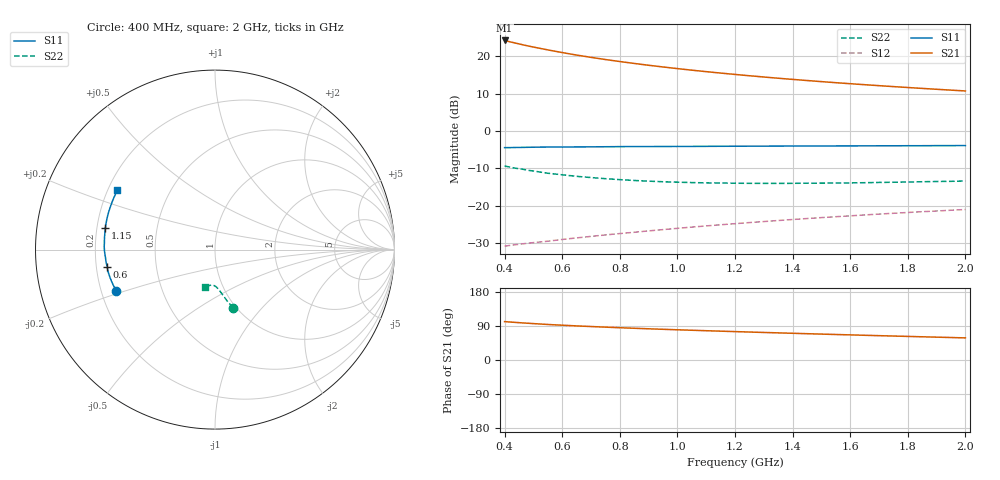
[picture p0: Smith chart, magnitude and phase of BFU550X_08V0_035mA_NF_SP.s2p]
! Filename:  P:\Prog\Test\Noise\ATS_data\Testdata_Net\BFU550X attenuator noise\BFU550X_APG2013_44_C05_08p0V_035mA_NF_CM01_D.sf
! Date/Time: Fri 26/Jul/2013 14:34:24
! BFU550X_APG2013_44_C05_08p0V_1to35mA_NF_CM01_Bias8_R.sf
! Noise Parameter Data File
! BFU550X_APG2013_44_C05_08p0V_1to35mA_NF_CM01
! Date/time: Mon Jul 22 10:19:05 2013
! VAR V_out= 8.001000
! VAR I_out= 34.995000
! VAR V_in= 0.782000
! VAR I_in= 0.370650
! Device data file deembeded for feedlines and parallel
! Original file: \BFU550X attenuator noise\BFU550X_APG2013_44_C05_08p0V_035mA_NF_CM01_R.sf
! Feed-files: PR005V01_100713_Feed1.s2p, PR005V01_100713_Feed2.s2p
! Parallel-file: PR005V01_100713_Par.s2p
# MHz S MA R 50
!  Freq-MHz  S11-mag  S11-arg  S21-mag  S21-arg  S12-mag  S12-arg  S22-mag  S22-arg
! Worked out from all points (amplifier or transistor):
!   37 points, 400 MHz to 2 GHz, reference 50 ohm
!   highest |S21| = 24.2 dB at 400 MHz (marker M1)
!   |S21| within 3 dB of that: start of sweep to 583.3 MHz
!   unconditionally stable (mu >= 1): 1.217 GHz to end of sweep
!   at 500 MHz: K = 0.74, MSG = 26.2 dB, |S12| = -29.9 dB
!   at 1.1 GHz: K = 0.98, MSG = 20.6 dB, |S12| = -25.4 dB
!   at 2 GHz: K = 1.05, MAG = 14.5 dB, |S12| = -21.0 dB
!   lowest NFmin = 1.31 dB at 480 MHz
!   S11 on the Smith chart (normalised r, x): 400 MHz: 0.26, -0.19; 600 MHz: 0.25, -0.07; 1.15 GHz: 0.23, +0.09; 2 GHz: 0.24, +0.27
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400  0.597 -157.4  16.2 101.3  0.02873 50.4  0.3391 -72.8
420  0.5974 -159.1  15.5 100.1  0.02947 50.8  0.3269 -73.9
440  0.6003 -160.7  14.87 99.1  0.03015 51.0  0.3158 -74.5
460  0.6017 -162.2  14.28 98.0  0.0308 51.3  0.3085 -75.6
480  0.6033 -163.6  13.72 97.0  0.03142 51.6  0.2978 -76.4
500  0.6053 -165.0  13.22 96.0  0.03205 51.9  0.2907 -77.0
550  0.6083 -168.4  12.12 93.7  0.03346 53.1  0.2715 -78.7
600  0.6082 -170.9  11.16 91.8  0.03531 53.9  0.2587 -80.1
650  0.6108 -173.4  10.34 90.0  0.03707 54.7  0.2469 -81.3
700  0.6116 -175.7  9.628 88.3  0.0388 55.5  0.2376 -82.6
750  0.614 -177.8  9.008 86.7  0.04062 56.2  0.2297 -83.7
800  0.6161 -179.7  8.467 85.2  0.04235 56.8  0.2228 -84.9
900  0.6173 176.6  7.548 82.4  0.04599 58.1  0.2127 -86.9
950  0.6187 174.9  7.163 81.0  0.04784 58.5  0.2089 -87.8
1050  0.6203 171.8  6.491 78.5  0.05169 59.4  0.2036 -89.6
1150  0.6226 169.0  5.935 76.1  0.05553 59.9  0.2009 -91.3
1200  0.6236 167.5  5.692 74.9  0.05742 60.1  0.1997 -92.2
1350  0.6264 163.5  5.064 71.6  0.06329 60.6  0.1985 -94.6
1500  0.6288 159.8  4.562 68.4  0.06923 60.8  0.2001 -97.0
1600  0.6302 157.4  4.278 66.3  0.07311 60.8  0.2017 -98.4
1750  0.6323 153.9  3.912 63.2  0.07909 60.6  0.2057 -100.8
2000  0.6369 148.6  3.42 58.3  0.08889 60.2  0.2137 -104.4
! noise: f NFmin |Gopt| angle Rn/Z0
400  1.387  0.355  -172.9  0.0873
460  1.346  0.4033  -172.1  0.0692
600  1.355  0.3928  -170.1  0.0754
800  1.377  0.4234  -166.7  0.069
1000  1.369  0.4519  -163.6  0.0656
1200  1.422  0.462  -160.1  0.0682
1400  1.456  0.4746  -157.4  0.0711
1600  1.483  0.4947  -151.9  0.0791
1800  1.505  0.4724  -150.9  0.0887
2000  1.534  0.4518  -146.6  0.1156
